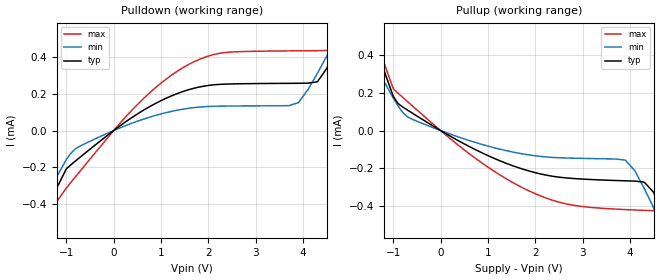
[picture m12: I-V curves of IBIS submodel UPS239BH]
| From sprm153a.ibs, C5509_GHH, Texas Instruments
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| Submodel   UPS239BH
[SubModel]   UPS239BH
 Submodel_type   Bus_hold
[Submodel Spec]
|Subparameter   typ   min   max
V_trigger_r   1.34   1.23   1.48
V_trigger_f   1.74   1.60   1.89
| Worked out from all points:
|   slope of the pulldown table from 0 to 0.3 V, typ, clamps not added: 5.33 kohm
|   slope of the pullup table from 0 to 0.3 V, typ, clamps not added: 6.93 kohm
[Pulldown]
|Voltage   I(typ)   I(min)   I(max)
-3.3V     -2.289mA   -1.418mA   -3.199mA
-1.8V     -842.8uA   -568.4uA   -1.113mA
-1.4V     -477.6uA   -353.2uA   -589.7uA
-1.2V     -311.8uA   -250.7uA   -387uA
-900mV    -186uA     -121.8uA   -281.7uA
600mV     106.5uA    59.75uA    167.5uA
1.75V     234.3uA    126.7uA    382.2uA
3.9V      258uA      152.4uA    435.3uA
4.3V      266uA      312.8uA    436uA
4.9V      653.7uA    600uA      514.8uA
5.1V      821.2uA    697.4uA    729.7uA
6.6V      2.097mA    1.427mA    2.607mA
[Pullup]
|Voltage   I(typ)   I(min)   I(max)
-3.3V     2.096mA    1.281mA    2.984mA
-1.8V     817.1uA    549.4uA    1.088mA
-1.4V     481.1uA    355.9uA    592.1uA
-1.2V     319.8uA    261.3uA    360.1uA
-900mV    142.5uA    129.9uA    197.1uA
100mV     -14.75uA   -9.309uA   -21.22uA
1.95V     -218.9uA   -131.5uA   -327.6uA
3.9V      -264.9uA   -156uA     -416.5uA
4.5V      -326uA     -408.6uA   -422.7uA
4.9V      -660uA     -624.8uA   -492.1uA
5.1V      -844.4uA   -735.4uA   -720.4uA
6.6V      -2.289mA   -1.593mA   -2.776mA
[Ramp]
|Variable   typ   min   max
 dV/dt_r   0.06V/0.040ns   0.05V/0.080ns   0.10V/0.040ns
 dV/dt_f   0.08V/0.120ns   0.05V/0.180ns   0.13V/0.080ns
 R_load =  500
